FUNCTION_BLOCK MIS_ProfilePosition
VAR_INPUT
	eCmd : eCommand;
	bChangeEmidiatly : BOOL;
	rVelocityRpm : REAL; //
	rAccellRpms : REAL; //
	lrTargetPos : LREAL;//
	
END_VAR
VAR_IN_OUT
	stMisMotorLocal : stMisMotor;	
END_VAR
VAR_OUTPUT
	eError : eErrorCodesMIS;
	eStat: ESTATUS;
END_VAR
VAR
	iState : INT;
	bInposition : BOOL;
	bSetPoint : BOOL;	
	bSetpointAwk: BOOL;
	
	SDO_WRITE : SDOwrite;
	WriteError: DWORD;
 	WriteData:ARRAY[0..255] OF BYTE;

END_VAR

IF eCmd = eCommand.Reset THEN
	eError := eErrorCodesMIS.None;
	iState := 0;
	eStat := eStatus.Done;
	RETURN;
END_IF;

//Read status word bits
bInposition := ((stMisMotorLocal.uiStatus AND 16#400) > 0);
bSetpointAwk := ((stMisMotorLocal.uiStatus AND 16#1000) > 0);



CASE iState OF 
0:
	CASE eCmd OF
	eCommand.Run:
		eStat := eStatus.Running;
		eError := eErrorCodesMIS.None;
		iState := 100;
	END_CASE

100: 
	stMisMotorLocal.diTargetpos := ANY_TO_DINT(lrTargetPos * stMisMotorLocal.lrUnitConversion);
	stMisMotorLocal.udiProfileVel := ANY_TO_UDINT(rVelocityRpm * ANY_TO_REAL(stMisMotorLocal.diRpmConversion));
	stMisMotorLocal.udiTargetAccel := ANY_TO_UDINT(rAccellRpms);
	iState := 130; 
	

130: //Wait for prior setpoint reset 
	bSetPoint := FALSE;	
	IF NOT bSetpointAwk THEN 
		iState := iState + 1;
	END_IF;

131://start motion
	bSetPoint := TRUE;	
	IF bSetpointAwk THEN 
		bSetPoint := FALSE;	
		bChangeEmidiatly := FALSE;
		eStat := eStatus.CmdOk; //Command completed
		iState := iState + 1;
	END_IF;	

132: //Wait for inposition 
	IF eCmd = eCommand.Stop THEN
		iState := 900; //Quickstop			
	ELSIF bInposition THEN
		iState := 1000; //Inposition / Done
	END_IF	
	
900: //Quick stop
	stMisMotorLocal.bQuickStop := TRUE;
	IF stMisMotorLocal.State = eDSP402States.QUICK_STOP_ACTIVE THEN
		stMisMotorLocal.bQuickStop := FALSE;
		iState := 1000;
	END_IF
	
1000:
	eStat := eStatus.Done;
	IF eCmd <> eCommand.Run THEN 
		iState := 0;		
	END_IF
	
END_CASE;


//Set controlword bits
stMisMotorLocal.uiCtrWord := ANY_TO_UINT(CSETBIT32(inVal32 := stMisMotorLocal.uiCtrWord,bitNo := 4,bitVal := bSetPoint));
stMisMotorLocal.uiCtrWord := ANY_TO_UINT(CSETBIT32(inVal32 := stMisMotorLocal.uiCtrWord,bitNo := 5,bitVal := bChangeEmidiatly));

END_FUNCTION_BLOCK
